| TEXAS INSTRUMENTS INCORPORATED
| Standard Linear and Logic Group
| IBIS Model of SN74AHC573
| OCTAL TRANSPERANT D-TYPE LATCHES WITH 3-STATE OUTPUTS
| This file contains package information for the following:
|  PDIP 20-pin (N) package as [Component] AHC573_N
|  SOIC 20-pin (DW) package as [Component] AHC573_DW
|  SOP 20-pin (NS) package as [Component] AHC573_NS
|  SSOP 20-pin (DB) package as [Component] AHC573_DB
|  TSSOP 20-pin (PW) package as [Component] AHC573_PW
|  TVSOP 20-pin (DGV) package as [Component] AHC573_DGV
| This device can be powered at the following Vccs:
|  5 volt Vcc
|  3.3 volt Vcc
|  2.5 volt Vcc
| This file provides unique models under the [Model Selector] for each Vcc.
| For operation at a specific Vcc, select the appropriate model after each
| [Model Selector] keyword.
[IBIS Ver]   3.2
[Comment char]  |_char
[File Name]   sn74ahc573.ibs
[File Rev]   1 | a_die
[Date]   December 1, 2021
[Source]   Data created from TI-SPICE simulations at TI-SLL.
[Notes]   Created from SN74AHC373 IBIS file
[Disclaimer] Property of Texas Instruments Incorporated.  Unauthorized
   reproduction and/or distribution is strictly prohibited.
   This product is protected under copyright law.
   Created  2006, (C) Copyright  2006, Texas Instruments
   Incorporated, All Rights Reserved
   UNLESS THERE IS A SIGNED, WRITTEN AGREEMENT TO THE
   CONTRARY, TEXAS INSTRUMENTS (TI) IS PROVIDING THE IBIS
   MODELS  AND WITHOUT ANY WARRANTY, EXPRESSED OR
   IMPLIED.  TI assumes no liability for:
   1) the accuracy of the IBIS models provided to your
   company;
   2) the proper functioning of these IBIS Models in your
   design or for any resulting applications; or
   3) infringement of patents, copyrights or intellectual
   property rights resulting from your use of these IBIS
   models.
   TI provides IBIS Models as a service to our customers.
   You and your company shall not distribute, sell or give
   these models to anyone else without prior written
   permission from TI.
   TI reserves the right to make changes to our products or
   to discontinue any semiconductor product or service
   without notice, and advises our customers to obtain the
   latest version of relevant information to verify, before
   placing orders, that the information being relied on is
   current.
   Please be aware that your receipt and use of the IBIS
   information provided shall serve as acceptance of these
   terms and conditions.  If you do not accept these terms,
   you should return or destroy the IBIS models and any
   other accompanying information immediately.
| Component SN74AHC573_N 20-PIN PDIP
[Component]   SN74AHC573_N
[Manufacturer]   Texas Instruments, Inc.
[Package]
|   typ   min   max
R_pkg   4.300e-02   3.800e-02   5.000e-02
L_pkg   7.384e-09   4.680e-09   1.032e-08
C_pkg   5.100e-13   2.310e-13   8.210e-13
[Pin]   signal_name   model_name   R_pin   L_pin   C_pin
1   NOE   AHC573_OEN   4.200e-02   9.427e-09   8.100e-13
2   1D   AHC573_IN   4.800e-02   7.163e-09   4.350e-13
3   2D   AHC573_IN   4.000e-02   4.825e-09   2.610e-13
4   3D   AHC573_IN   4.000e-02   6.359e-09   4.890e-13
5   4D   AHC573_IN   3.800e-02   7.982e-09   4.750e-13
6   5D   AHC573_IN   3.800e-02   7.978e-09   4.760e-13
7   6D   AHC573_IN   4.000e-02   6.302e-09   4.920e-13
8   7D   AHC573_IN   4.000e-02   4.822e-09   2.610e-13
9   8D   AHC573_IN   4.700e-02   7.118e-09   4.390e-13
10   GND   GND   5.000e-02   1.032e-08   8.050e-13
11   LE   AHC573_LE   5.000e-02   1.028e-08   8.100e-13
12   8Q   AHC573_OUT   4.600e-02   8.492e-09   4.610e-13
13   7Q   AHC573_OUT   4.000e-02   5.284e-09   6.480e-13
14   6Q   AHC573_OUT   4.000e-02   4.680e-09   2.310e-13
15   5Q   AHC573_OUT   4.300e-02   9.383e-09   4.770e-13
16   4Q   AHC573_OUT   4.300e-02   9.403e-09   4.750e-13
17   3Q   AHC573_OUT   4.000e-02   4.686e-09   2.320e-13
18   2Q   AHC573_OUT   4.000e-02   5.284e-09   6.480e-13
19   1Q   AHC573_OUT   4.600e-02   8.544e-09   4.560e-13
20   VCC   POWER   4.300e-02   9.348e-09   8.210e-13
| Component SN74AHC573_DW 20-PIN SOIC
[Component]   SN74AHC573_DW
[Manufacturer]   Texas Instruments, Inc.
[Package]
|   typ   min   max
R_pkg   3.800e-02   3.300e-02   4.500e-02
L_pkg   5.012e-09   4.110e-09   6.349e-09
C_pkg   7.170e-13   5.300e-13   8.680e-13
[Pin]   signal_name   model_name   R_pin   L_pin   C_pin
1   NOE   AHC573_OEN   4.200e-02   9.427e-09   8.100e-13
2   1D   AHC573_IN   4.800e-02   7.163e-09   4.350e-13
3   2D   AHC573_IN   4.000e-02   4.825e-09   2.610e-13
4   3D   AHC573_IN   4.000e-02   6.359e-09   4.890e-13
5   4D   AHC573_IN   3.800e-02   7.982e-09   4.750e-13
6   5D   AHC573_IN   3.800e-02   7.978e-09   4.760e-13
7   6D   AHC573_IN   4.000e-02   6.302e-09   4.920e-13
8   7D   AHC573_IN   4.000e-02   4.822e-09   2.610e-13
9   8D   AHC573_IN   4.700e-02   7.118e-09   4.390e-13
10   GND   GND   5.000e-02   1.032e-08   8.050e-13
11   LE   AHC573_LE   5.000e-02   1.028e-08   8.100e-13
12   8Q   AHC573_OUT   4.600e-02   8.492e-09   4.610e-13
13   7Q   AHC573_OUT   4.000e-02   5.284e-09   6.480e-13
14   6Q   AHC573_OUT   4.000e-02   4.680e-09   2.310e-13
15   5Q   AHC573_OUT   4.300e-02   9.383e-09   4.770e-13
16   4Q   AHC573_OUT   4.300e-02   9.403e-09   4.750e-13
17   3Q   AHC573_OUT   4.000e-02   4.686e-09   2.320e-13
18   2Q   AHC573_OUT   4.000e-02   5.284e-09   6.480e-13
19   1Q   AHC573_OUT   4.600e-02   8.544e-09   4.560e-13
20   VCC   POWER   4.300e-02   9.348e-09   8.210e-13
| Component SN74AHC573_NS 20-PIN SOP
[Component]   SN74AHC573_NS
[Manufacturer]   Texas Instruments, Inc.
[Package]
|   typ   min   max
R_pkg   4.400e-02   2.900e-02   5.800e-02
L_pkg   3.666e-09   2.317e-09   5.115e-09
C_pkg   5.480e-13   3.160e-13   7.250e-13
[Pin]   signal_name   model_name   R_pin   L_pin   C_pin
1   NOE   AHC573_OEN   4.200e-02   9.427e-09   8.100e-13
2   1D   AHC573_IN   4.800e-02   7.163e-09   4.350e-13
3   2D   AHC573_IN   4.000e-02   4.825e-09   2.610e-13
4   3D   AHC573_IN   4.000e-02   6.359e-09   4.890e-13
5   4D   AHC573_IN   3.800e-02   7.982e-09   4.750e-13
6   5D   AHC573_IN   3.800e-02   7.978e-09   4.760e-13
7   6D   AHC573_IN   4.000e-02   6.302e-09   4.920e-13
8   7D   AHC573_IN   4.000e-02   4.822e-09   2.610e-13
9   8D   AHC573_IN   4.700e-02   7.118e-09   4.390e-13
10   GND   GND   5.000e-02   1.032e-08   8.050e-13
11   LE   AHC573_LE   5.000e-02   1.028e-08   8.100e-13
12   8Q   AHC573_OUT   4.600e-02   8.492e-09   4.610e-13
13   7Q   AHC573_OUT   4.000e-02   5.284e-09   6.480e-13
14   6Q   AHC573_OUT   4.000e-02   4.680e-09   2.310e-13
15   5Q   AHC573_OUT   4.300e-02   9.383e-09   4.770e-13
16   4Q   AHC573_OUT   4.300e-02   9.403e-09   4.750e-13
17   3Q   AHC573_OUT   4.000e-02   4.686e-09   2.320e-13
18   2Q   AHC573_OUT   4.000e-02   5.284e-09   6.480e-13
19   1Q   AHC573_OUT   4.600e-02   8.544e-09   4.560e-13
20   VCC   POWER   4.300e-02   9.348e-09   8.210e-13
| Component SN74AHC573_DB 20-PIN SSOP
[Component]   SN74AHC573_DB
[Manufacturer]   Texas Instruments, Inc.
[Package]
|   typ   min   max
R_pkg   4.000e-02   3.500e-02   5.100e-02
L_pkg   3.495e-09   3.035e-09   4.314e-09
C_pkg   4.200e-13   3.460e-13   5.020e-13
[Pin]   signal_name   model_name   R_pin   L_pin   C_pin
1   NOE   AHC573_OEN   4.200e-02   9.427e-09   8.100e-13
2   1D   AHC573_IN   4.800e-02   7.163e-09   4.350e-13
3   2D   AHC573_IN   4.000e-02   4.825e-09   2.610e-13
4   3D   AHC573_IN   4.000e-02   6.359e-09   4.890e-13
5   4D   AHC573_IN   3.800e-02   7.982e-09   4.750e-13
6   5D   AHC573_IN   3.800e-02   7.978e-09   4.760e-13
7   6D   AHC573_IN   4.000e-02   6.302e-09   4.920e-13
8   7D   AHC573_IN   4.000e-02   4.822e-09   2.610e-13
9   8D   AHC573_IN   4.700e-02   7.118e-09   4.390e-13
10   GND   GND   5.000e-02   1.032e-08   8.050e-13
11   LE   AHC573_LE   5.000e-02   1.028e-08   8.100e-13
12   8Q   AHC573_OUT   4.600e-02   8.492e-09   4.610e-13
13   7Q   AHC573_OUT   4.000e-02   5.284e-09   6.480e-13
14   6Q   AHC573_OUT   4.000e-02   4.680e-09   2.310e-13
15   5Q   AHC573_OUT   4.300e-02   9.383e-09   4.770e-13
16   4Q   AHC573_OUT   4.300e-02   9.403e-09   4.750e-13
17   3Q   AHC573_OUT   4.000e-02   4.686e-09   2.320e-13
18   2Q   AHC573_OUT   4.000e-02   5.284e-09   6.480e-13
19   1Q   AHC573_OUT   4.600e-02   8.544e-09   4.560e-13
20   VCC   POWER   4.300e-02   9.348e-09   8.210e-13
| Component SN74AHC573_PW 20-PIN TSSOP
[Component]   SN74AHC573_PW
[Manufacturer]   Texas Instruments, Inc.
[Package]
|   typ   min   max
R_pkg   5.000e-02   4.200e-02   6.000e-02
L_pkg   2.802e-09   2.248e-09   3.553e-09
C_pkg   3.170e-13   2.020e-13   4.430e-13
[Pin]   signal_name   model_name   R_pin   L_pin   C_pin
1   NOE   AHC573_OEN   4.200e-02   9.427e-09   8.100e-13
2   1D   AHC573_IN   4.800e-02   7.163e-09   4.350e-13
3   2D   AHC573_IN   4.000e-02   4.825e-09   2.610e-13
4   3D   AHC573_IN   4.000e-02   6.359e-09   4.890e-13
5   4D   AHC573_IN   3.800e-02   7.982e-09   4.750e-13
6   5D   AHC573_IN   3.800e-02   7.978e-09   4.760e-13
7   6D   AHC573_IN   4.000e-02   6.302e-09   4.920e-13
8   7D   AHC573_IN   4.000e-02   4.822e-09   2.610e-13
9   8D   AHC573_IN   4.700e-02   7.118e-09   4.390e-13
10   GND   GND   5.000e-02   1.032e-08   8.050e-13
11   LE   AHC573_LE   5.000e-02   1.028e-08   8.100e-13
12   8Q   AHC573_OUT   4.600e-02   8.492e-09   4.610e-13
13   7Q   AHC573_OUT   4.000e-02   5.284e-09   6.480e-13
14   6Q   AHC573_OUT   4.000e-02   4.680e-09   2.310e-13
15   5Q   AHC573_OUT   4.300e-02   9.383e-09   4.770e-13
16   4Q   AHC573_OUT   4.300e-02   9.403e-09   4.750e-13
17   3Q   AHC573_OUT   4.000e-02   4.686e-09   2.320e-13
18   2Q   AHC573_OUT   4.000e-02   5.284e-09   6.480e-13
19   1Q   AHC573_OUT   4.600e-02   8.544e-09   4.560e-13
20   VCC   POWER   4.300e-02   9.348e-09   8.210e-13
| Component SN74AHC573_DGV 20-PIN TVSOP
[Component]   SN74AHC573_DGV
[Manufacturer]   Texas Instruments, Inc.
[Package]
|   typ   min   max
R_pkg   4.400e-02   3.800e-02   4.800e-02
L_pkg   2.561e-09   2.236e-09   2.961e-09
C_pkg   3.420e-13   2.640e-13   4.460e-13
[Pin]   signal_name   model_name   R_pin   L_pin   C_pin
1   NOE   AHC573_OEN   4.200e-02   9.427e-09   8.100e-13
2   1D   AHC573_IN   4.800e-02   7.163e-09   4.350e-13
3   2D   AHC573_IN   4.000e-02   4.825e-09   2.610e-13
4   3D   AHC573_IN   4.000e-02   6.359e-09   4.890e-13
5   4D   AHC573_IN   3.800e-02   7.982e-09   4.750e-13
6   5D   AHC573_IN   3.800e-02   7.978e-09   4.760e-13
7   6D   AHC573_IN   4.000e-02   6.302e-09   4.920e-13
8   7D   AHC573_IN   4.000e-02   4.822e-09   2.610e-13
9   8D   AHC573_IN   4.700e-02   7.118e-09   4.390e-13
10   GND   GND   5.000e-02   1.032e-08   8.050e-13
11   LE   AHC573_LE   5.000e-02   1.028e-08   8.100e-13
12   8Q   AHC573_OUT   4.600e-02   8.492e-09   4.610e-13
13   7Q   AHC573_OUT   4.000e-02   5.284e-09   6.480e-13
14   6Q   AHC573_OUT   4.000e-02   4.680e-09   2.310e-13
15   5Q   AHC573_OUT   4.300e-02   9.383e-09   4.770e-13
16   4Q   AHC573_OUT   4.300e-02   9.403e-09   4.750e-13
17   3Q   AHC573_OUT   4.000e-02   4.686e-09   2.320e-13
18   2Q   AHC573_OUT   4.000e-02   5.284e-09   6.480e-13
19   1Q   AHC573_OUT   4.600e-02   8.544e-09   4.560e-13
20   VCC   POWER   4.300e-02   9.348e-09   8.210e-13
| Model AHC573_LE
[Model Selector]   AHC573_LE
AHC573_LE_50   5 volt Vcc
AHC573_LE_33   3.3 volt Vcc
AHC573_LE_25   2.5 volt Vcc
| Model AHC573_IN
[Model Selector]   AHC573_IN
AHC573_IN_50   5 volt Vcc
AHC573_IN_33   3.3 volt Vcc
AHC573_IN_25   2.5 volt Vcc
| Model AHC573_OEN
[Model Selector]   AHC573_OEN
AHC573_OEN_50   5 volt Vcc
AHC573_OEN_33   3.3 volt Vcc
AHC573_OEN_25   2.5 volt Vcc
| Model AHC573_OUT
[Model Selector]   AHC573_OUT
AHC573_OUT_50   5 volt Vcc
AHC573_OUT_33   3.3 volt Vcc
AHC573_OUT_25   2.5 volt Vcc
| Models and submodels in the file (12): AHC573_LE_50 (Input), AHC573_LE_33 (Input), AHC573_LE_25 (Input), AHC573_IN_50 (Input), AHC573_IN_33 (Input), AHC573_IN_25 (Input), AHC573_OEN_50 (Input), AHC573_OEN_33 (Input), AHC573_OEN_25 (Input), AHC573_OUT_50 (3-state), AHC573_OUT_33 (3-state), AHC573_OUT_25 (3-state)
